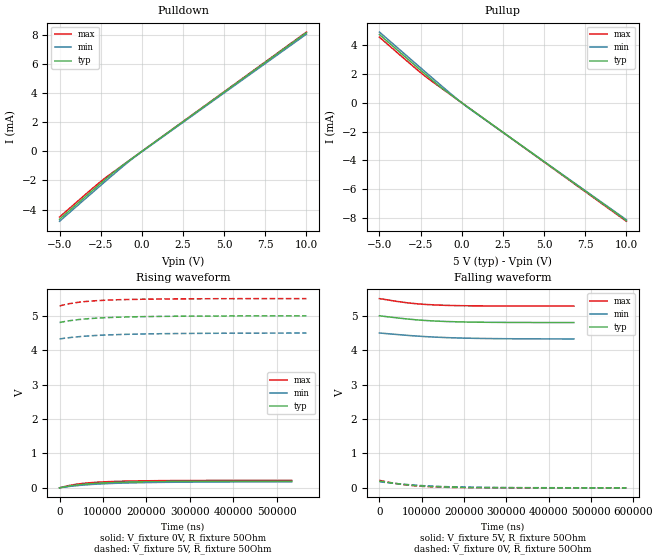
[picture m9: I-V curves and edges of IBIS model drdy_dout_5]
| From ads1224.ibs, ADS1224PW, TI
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|   drdy_dout_5 Model
[Model]   drdy_dout_5
Model_type   Output
Polarity   Non-Inverting
Vmeas = 2.5
Vref = 2.5
Cref = 2pF
Rref = 50
|   typ   min   max
|   (nom PVT)   (fast PVT)   (slow PVT)
|C_comp from frequency sweep method (F= 2.5MHz)
|Average
|C_comp   8.43e-15   7.16e-15   1.01e-14
|ON state : BUFFER OUTPUT TURNED HIGH
C_comp   6.356e-15   5.378e-15   7.602e-15
|OFF state: BUFFER IN HIGH IMPEDANCE
|C_comp   1.050e-14   8.933e-15   1.266e-14
|C_comp from LC tank measurement(L=1nH)
|Average
|Resonant Frequency(Hz)  1.000e+12   1.000e+12   1.000e+12
|C_comp   2.536e-17   2.536e-17   2.536e-17
|ON state : BUFFER OUTPUT TURNED HIGH
|Resonant Frequency(Hz)  1.000e+12   1.000e+12   1.000e+12
|C_comp   2.536e-17   2.536e-17   2.536e-17
|OFF state: BUFFER IN HIGH IMPEDANCE
|Resonant Frequency(Hz)  1.000e+12   1.000e+12   1.000e+12
|C_comp   2.536e-17   2.536e-17   2.536e-17
| Where nom  PVT is Nominal Process, 5V, 25C
|   Fast PVT is Strong Process,  5.5V, -40C
|   Slow PVT is Weak Process,   4.5V, 85C
[Voltage Range]   5   4.5   5.5
|Ambient Temperature   25   85   -40
|Junction Temperature
[Temperature Range]   25   85   -40
[Pullup Reference]   5   4.5   5.5
[Pulldown Reference]   0   0   0
[Power Clamp Reference]   5   4.5   5.5
[GND Clamp Reference]   0   0   0
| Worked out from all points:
|   slope of the pulldown table from 0 to 0.75 V, typ, clamps not added: 1.22 kohm
|   slope of the pullup table from 0 to 0.75 V, typ, clamps not added: 1.22 kohm
|   falling waveform, V_fixture 5V, R_fixture 50Ohm: 20-80 % time 114us typ, 137us min, 92.5us max; typ from 5 V to 4.8 V
|   rising waveform, V_fixture 0V, R_fixture 50Ohm: 20-80 % time 109us typ, 132us min, 89us max; typ from 0 V to 0.195 V
|   rising waveform, V_fixture 5V, R_fixture 50Ohm: 20-80 % time 121us typ, 144us min, 98.8us max; typ from 4.8 V to 5 V
|   falling waveform, V_fixture 0V, R_fixture 50Ohm: 20-80 % time 104us typ, 126us min, 84.9us max; typ from 0.196 V to 0 V
[Pulldown]
|   Voltage   I(typ)   I(min)   I(max)
-5V       -4.666mA   -4.807mA   -4.515mA
-2.36V    -2.064mA   -2.2mA     -1.947mA
-1.25V    -1.027mA   -1.125mA   -1.023mA
0V        0A         0A         0A
10V       8.175mA    8.075mA    8.215mA
[Pullup]
|   Voltage   I(typ)   I(min)   I(max)
-5V       4.723mA    4.892mA    4.539mA
-2.256V   2.012mA    2.174mA    1.862mA
-1.25V    1.049mA    1.187mA    1.021mA
314.5mV   -260.1uA   -288uA     -262.2uA
10V       -8.154mA   -8.106mA   -8.21mA
[Ramp]
R_load = 50
|   typ   min   max
dV/dt_r   0.11744/0.00010999   0.104791/0.000135006   0.13/8.92752e-05
dV/dt_f   0.117741/0.000114094   0.104263/0.00013985   0.130088/9.26212e-05
[Falling Waveform]
V_fixture = 5V
V_fixture_min = 4.5V
V_fixture_max = 5.5V
R_fixture = 50Ohm
|   Time   V(typ)   V(min)   V(max)
0s        5V         4.5V       5.5V
38.01us   4.945V     4.46V      5.425V
70.88us   4.902V     4.427V     5.371V
89.4us    4.882V     4.411V     5.349V
110.4us   4.863V     4.395V     5.329V
134.6us   4.846V     4.379V     5.314V
194.5us   4.822V     4.353V     5.294V
239.6us   4.814V     4.342V     5.288V
334.2us   4.806V     4.331V     5.284V
460us     4.804V     4.327V     5.283V
[Rising Waveform]
V_fixture = 0V
V_fixture_min = 0V
V_fixture_max = 0V
R_fixture = 50Ohm
|   Time   V(typ)   V(min)   V(max)
0s        35.75uV    1.494mV    37.52uV
11.09us   27.4mV     21.42mV    37.4mV
22.13us   51.1mV     39.12mV    68.47mV
38.01us   78.76mV    60.95mV    103.2mV
53.99us   101.1mV    80.37mV    128.9mV
89.4us    135.3mV    109.7mV    165.1mV
134.6us   160.2mV    133.8mV    189.1mV
194.5us   177.3mV    151.8mV    203.9mV
284.2us   188.3mV    165mV      212.4mV
534.2us   195.1mV    174.7mV    216.5mV
[Rising Waveform]
V_fixture = 5V
V_fixture_min = 4.5V
V_fixture_max = 5.5V
R_fixture = 50Ohm
|   Time   V(typ)   V(min)   V(max)
0s        4.804V     4.326V     5.283V
11.09us   4.832V     4.347V     5.321V
22.13us   4.855V     4.364V     5.351V
38.01us   4.881V     4.385V     5.383V
53.99us   4.902V     4.403V     5.408V
89.4us    4.935V     4.431V     5.442V
134.6us   4.959V     4.454V     5.466V
194.5us   4.976V     4.472V     5.482V
284.2us   4.988V     4.486V     5.492V
568.2us   4.999V     4.499V     5.499V
[Falling Waveform]
V_fixture = 0V
V_fixture_min = 0V
V_fixture_max = 0V
R_fixture = 50Ohm
|   Time   V(typ)   V(min)   V(max)
0s        195.8mV    176.1mV    216.7mV
38.01us   128.3mV    126.1mV    127.1mV
53.99us   104.8mV    107mV      98.1mV
70.88us   83.59mV    89.98mV    73.71mV
89.4us    64.63mV    73.72mV    53.48mV
110.4us   48mV       58.27mV    37.01mV
134.6us   33.94mV    44.24mV    24.2mV
194.5us   14.33mV    22.71mV    8.564mV
284.2us   4.21mV     8.855mV    1.929mV
584.2us   97.38uV    1.728mV    46.76uV
